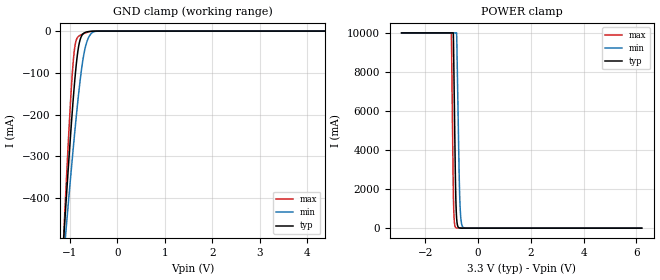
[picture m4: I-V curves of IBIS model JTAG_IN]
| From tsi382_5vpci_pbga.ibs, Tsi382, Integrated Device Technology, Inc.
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|   MODEL JTAG_IN
[Model]   JTAG_IN
Model_type  Input
C_comp 2.388p 2.203p 2.58p
Polarity   Non-Inverting
Enable   Active-High
|   typ   min   max
Vinl   =   0.800v
Vinh   =   2.000v
[Model Spec]
[Temperature Range]   25   125   -40
[Voltage Range] 3.3 3.135 3.465
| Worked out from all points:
|   GND clamp passes 1 mA (typ) near -0.60 V on its own axis
|   POWER clamp passes 1 mA (typ) near -0.61 V on its own axis
[GND Clamp]
-2.907V   -3.934A    -3.096A    -5.193A
-1.131V   -496.2mA   -541.1mA   -489.3mA
-1.119V   -474.7mA   -524.9mA   -460.4mA
-1.083V   -410.9mA   -476.5mA   -375mA
-986.3mV  -248mA     -350.5mA   -166mA
-913.9mV  -138.9mA   -260.3mA   -52.82mA
-877.6mV  -92.52mA   -217.3mA   -25.74mA
-817.2mV  -36.84mA   -150.4mA   -12.5mA
-696.5mV  -4.247mA   -49.47mA   -5.397mA
-587.8mV  -839.7uA   -11.35mA   -1.556mA
-442.9mV  -58.38uA   -420.2uA   -88.72uA
4.367V    0A         0A         0A
[Power Clamp]
-2.907V   10A        10A        10A
-1.016V   10A        10A        10A
-946.5mV  10A        10A        2.16A
-934.9mV  9.361A     10A        1.335A
-905.8mV  6.537A     10A        358.9mA
-847.7mV  1.488A     10A        27.56mA
-812.8mV  425mA      9.727A     9.595mA
-725.5mV  17.06mA    3.032A     3.852mA
-696.4mV  6.59mA     1.448A     3.168mA
-649.9mV  1.96mA     402mA      2.225mA
-580.1mV  566.8uA    54.17mA    1.101mA
6.207V    0A         0A         0A
